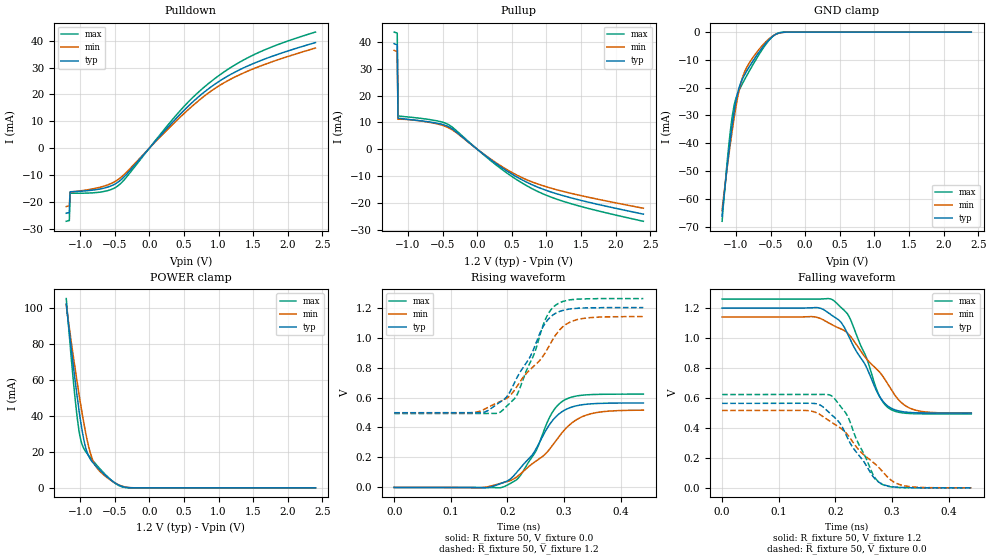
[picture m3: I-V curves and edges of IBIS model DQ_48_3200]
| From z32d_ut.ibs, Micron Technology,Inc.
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| MODEL DQ_48_3200 (48 Ohm Data I/O with no ODT, 1600-3200Mbps)
[Model]   DQ_48_3200
Model_type   I/O
Vinl = 905.000mV
Vinh = 1015.000mV
Vmeas = 960.000mV
Vref = 1200.000mV
Cref = 0.0pF
Rref = 50.000Ohm
|   typ   min   max
|C_comp   0.636pF   0.586pF   0.686pF
C_comp_pullup   0.318pF   0.293pF   0.343pF
C_comp_pulldown   0.318pF   0.293pF   0.343pF
[Model Spec]
| Timing spec test load voltage corners
Vref   1.2000V   1.1400V   1.2600V
| Dynamic Overshoot Parameters from DDR4 Specification
|D_overshoot_ampl_h   0.40   NA   NA
|D_overshoot_ampl_l   0.40   NA   NA
|D_overshoot_area_h   0.0800n   NA   NA
|D_overshoot_area_l   0.0800n   NA   NA
[Voltage Range]   1.2000V   1.1400V   1.2600V
| Junction Temperature (Ambient temp is 35C typ, 125C min, -40C max)
[Temperature Range]   50.0   140.0   -40.0
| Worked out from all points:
|   slope of the pulldown table from 0 to 0.18 V, typ, clamps not added: 34.3 ohm
|   slope of the pullup table from 0 to 0.18 V, typ, clamps not added: 49.8 ohm
|   GND clamp passes 1 mA (typ) near -0.44 V on its own axis
|   POWER clamp passes 1 mA (typ) near -0.41 V on its own axis
|   rising waveform, R_fixture 50, V_fixture 0.0: 20-80 % time 61.7ps typ, 81.4ps min, 48.6ps max; typ from 0 V to 0.564 V
|   rising waveform, R_fixture 50, V_fixture 1.2: 20-80 % time 56.5ps typ, 76.1ps min, 45ps max; typ from 0.499 V to 1.2 V
|   falling waveform, R_fixture 50, V_fixture 1.2: 20-80 % time 56.4ps typ, 76.9ps min, 45.2ps max; typ from 1.2 V to 0.499 V
|   falling waveform, R_fixture 50, V_fixture 0.0: 20-80 % time 56.3ps typ, 80.9ps min, 43.6ps max; typ from 0.564 V to 0 V
[Pulldown]
|   Voltage   I(typ)   I(min)   I(max)
-1.2V     -24.27mA   -21.79mA   -27.26mA
-1.156V   -24mA      -21.51mA   -26.99mA
-1.145V   -16.26mA   -16.36mA   -16.8mA
-676.4mV  -15.03mA   -14.32mA   -16.25mA
-447.3mV  -12.57mA   -11.61mA   -13.91mA
-327.3mV  -9.698mA   -8.908mA   -10.71mA
425.5mV   12.1mA     11.05mA    13.4mA
643.6mV   17.6mA     16.21mA    19.29mA
927.3mV   23.48mA    21.9mA     25.55mA
1.2V      27.83mA    26.04mA    30.45mA
1.527V    31.8mA     29.83mA    35.03mA
2.4V      39.36mA    37.31mA    43.27mA
[GND Clamp]
|   Voltage   I(typ)   I(min)   I(max)
-1.2V     -66.16mA   -64.28mA   -68.09mA
-1.135V   -50.09mA   -50.4mA    -48.85mA
-1.091V   -40.54mA   -42.05mA   -37.85mA
-1.058V   -34.05mA   -36.16mA   -31.11mA
-1.015V   -26.75mA   -29.01mA   -25.14mA
-970.9mV  -21.46mA   -22.9mA    -21.88mA
-938.2mV  -18.78mA   -19.25mA   -20.13mA
-850.9mV  -14.3mA    -13.05mA   -15.99mA
-654.5mV  -6.796mA   -5.876mA   -7.607mA
-458.2mV  -1.354mA   -1.258mA   -1.328mA
-261.8mV  -15.07uA   -33uA      -1.874uA
2.4V      0A         0A         0A
[Pullup]
|   Voltage   I(typ)   I(min)   I(max)
-1.2V     39.44mA    36.96mA    43.78mA
-1.156V   39.03mA    36.52mA    43.4mA
-1.145V   11.61mA    11.2mA     12.43mA
-741.8mV  10.38mA    10.26mA    11.29mA
-425.5mV  8.536mA    8.147mA    9.339mA
-327.3mV  6.972mA    6.652mA    7.536mA
98.18mV   -1.997mA   -1.89mA    -2.176mA
414.5mV   -7.886mA   -7.401mA   -8.632mA
643.6mV   -11.37mA   -10.57mA   -12.55mA
938.2mV   -14.8mA    -13.53mA   -16.53mA
1.462V    -18.86mA   -17.1mA    -21.12mA
2.4V      -24.24mA   -22.03mA   -26.9mA
[POWER Clamp]
|   Voltage   I(typ)   I(min)   I(max)
-1.2V     102.5mA    102mA      105.3mA
-1.135V   79.77mA    83.1mA     75.19mA
-1.069V   58.73mA    65.56mA    48.4mA
-1.015V   42.76mA    51.76mA    31.44mA
-981.8mV  34.37mA    43.96mA    25.34mA
-905.5mV  20.47mA    27.87mA    19.42mA
-850.9mV  15.87mA    19.19mA    16.74mA
-807.3mV  13.63mA    14.48mA    14.72mA
-709.1mV  9.665mA    8.956mA    10.4mA
-501.8mV  2.9mA      2.85mA     2.745mA
-261.8mV  34uA       81.67uA    4.604uA
2.4V      0A         0A         0A
[Ramp]
|   typ   min   max
| 20% - 80%
dV/dt_r   338.19m/61.67p   309.42m/81.44p   373.57m/48.65p
dV/dt_f   420.87m/56.38p   384.89m/76.87p   460.07m/45.24p
| Slew rate: Power terminated
|SR_r[V/ns]   7.46   5.06   10.22
|SR_f[V/ns]   7.46   5.01   10.17
| 25% - 75%
|dV/dt_r   281.82m/49.79p   257.85m/67.02p   311.31m/39.25p
|dV/dt_f   350.73m/47.52p   320.74m/65.13p   383.39m/37.68p
| Slew rate: Power terminated
|SR_r[V/ns]   7.39   4.96   10.20
|SR_f[V/ns]   7.38   4.92   10.17
R_load = 50
[Rising Waveform]
R_fixture = 50
V_fixture = 0.0
|   Time   V(typ)   V(min)   V(max)
0s        6.769uV    38.78uV    398.2nV
162ps     -1.913mV   2.287mV    133.5uV
193ps     32.9mV     31.95mV    3.811mV
223ps     131.7mV    90.58mV    80.82mV
251ps     260.6mV    177.6mV    248.6mV
277ps     433.9mV    268.5mV    486.6mV
298ps     509.5mV    372.5mV    577.1mV
321ps     544.2mV    450mV      609.6mV
346ps     557.5mV    490.4mV    619.4mV
440ps     563.7mV    515.7mV    622.6mV
[Rising Waveform]
R_fixture   = 50
V_fixture   = 1.2
V_fixture_min = 1.14
V_fixture_max = 1.26
|   Time   V(typ)   V(min)   V(max)
0s        498.5mV    498.4mV    493.2mV
153ps     499mV      511mV      493.3mV
186ps     566.9mV    570.5mV    500.2mV
201ps     616.4mV    601.1mV    551.7mV
217ps     734.3mV    675.3mV    618.8mV
248ps     939.9mV    813.4mV    899.5mV
267ps     1.098V     900.6mV    1.122V
286ps     1.164V     1.023V     1.219V
325ps     1.196V     1.122V     1.257V
440ps     1.2V       1.14V      1.26V
[Falling Waveform]
R_fixture   = 50
V_fixture   = 1.2
V_fixture_min = 1.14
V_fixture_max = 1.26
|   Time   V(typ)   V(min)   V(max)
0s        1.2V       1.14V      1.26V
168ps     1.203V     1.137V     1.26V
193ps     1.153V     1.091V     1.259V
224ps     1.008V     1.023V     1.145V
255ps     804.3mV    860.9mV    867mV
275ps     629.7mV    785.3mV    635.9mV
292ps     547.6mV    696.2mV    538.7mV
313ps     512.2mV    581.9mV    503.4mV
336ps     501.9mV    524.9mV    495.2mV
440ps     498.5mV    498.5mV    493.2mV
[Falling Waveform]
R_fixture = 50
V_fixture = 0.0
|   Time   V(typ)   V(min)   V(max)
0s        563.7mV    516.4mV    622.6mV
162ps     563.4mV    508mV      622.6mV
191ps     495.2mV    442.7mV    618.5mV
208ps     431.6mV    401.7mV    548.8mV
220ps     344.5mV    361mV      489.3mV
265ps     83.15mV    176mV      100.1mV
280ps     30.02mV    122.7mV    29.53mV
299ps     8.139mV    49.69mV    6.176mV
321ps     1.825mV    14.2mV     1.01mV
440ps     7.785uV    56.56uV    515.6nV
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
